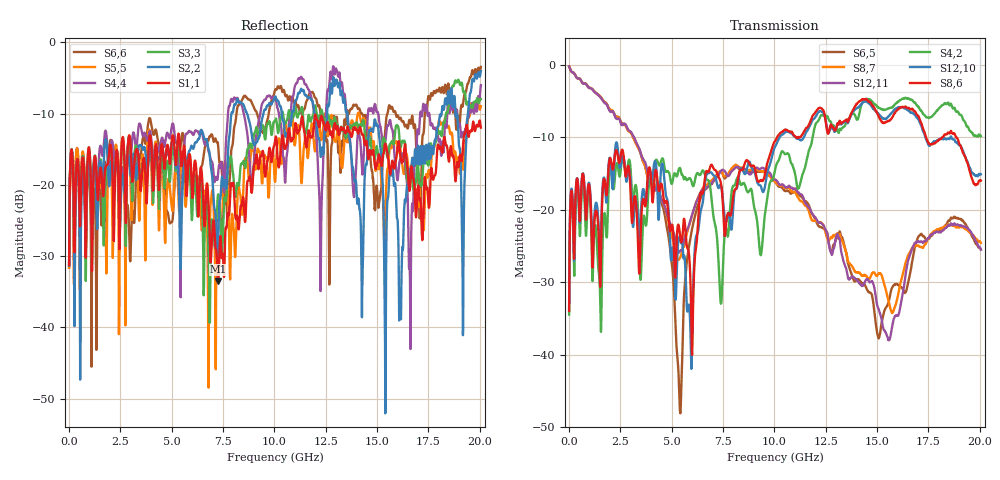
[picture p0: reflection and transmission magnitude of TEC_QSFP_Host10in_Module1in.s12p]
!!  This file represents Tyco Electronics parts only.  Due to internal design and materials, it should not  !!
!!  be used for products manufactured by companies other than Tyco Electronics.  !!
!! FILE NAME: TEC_QSFP_Host10in_Module1in.s12p
!! PART DESCRIPTION: Tyco Electronics QSFP P/N 1761987-9
!! PCB DESCRIPTION: Host Board FR4 with 10 inch microstrip, Module Board FR4 with 1.5 inch microstrip
!! FILE DESCRIPTION: 12 Port, S-Parameter, Measured Channel
!! FILE REVISION: Revision 1, 3/11/2008
!! FILE FREQUENCY RANGE: DC to 20.05 GHz in 12.50 MHz frequency steps
!! PORT DEFINITIONS:
!! Port  1  ----->  Host	Pin 14, RX3+	Module  <-----  Port  2
!! Port  3  ----->  Host	Pin 15, RX3-	Module  <-----  Port  4
!! Port  5  ----->  Host	Pin 21, RX2-	Module  <-----  Port  6
!! Port  7  ----->  Host	Pin 22, RX2+	Module  <-----  Port  8
!! Port  9  ----->  Host	Pin 24, RX4-	Module  <-----  Port  10
!! Port  11  ----->  Host	Pin 25, RX4+	Module  <-----  Port  12
# HZ S MA R 50.00
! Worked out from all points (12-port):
!   1604 points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, 12.5 MHz to 20.05 GHz, reference 50 ohm
!   strongest paths, dB at 12.5 MHz, 5.025 GHz, 10.04 GHz, 15.05 GHz, 20.05 GHz:
!     S8,6: -34.0, -22.1, -10.5, -6.9, -16.0
!     S12,10: -33.7, -26.0, -11.3, -6.7, -15.1
!     S4,2: -34.5, -16.4, -14.5, -5.9, -9.9
!     S12,11: -0.2, -22.7, -15.9, -33.6, -25.5
!     S8,7: -0.2, -23.8, -16.1, -28.9, -24.6
!     S6,5: -0.2, -27.8, -16.2, -37.5, -25.5
!   lowest |S11| = -33.5 dB at 7.263 GHz (marker M1), VSWR 1.04, Z = 48.7 + j1.63 ohm
!   |S11| at or under -10 dB: start of sweep to end of sweep
